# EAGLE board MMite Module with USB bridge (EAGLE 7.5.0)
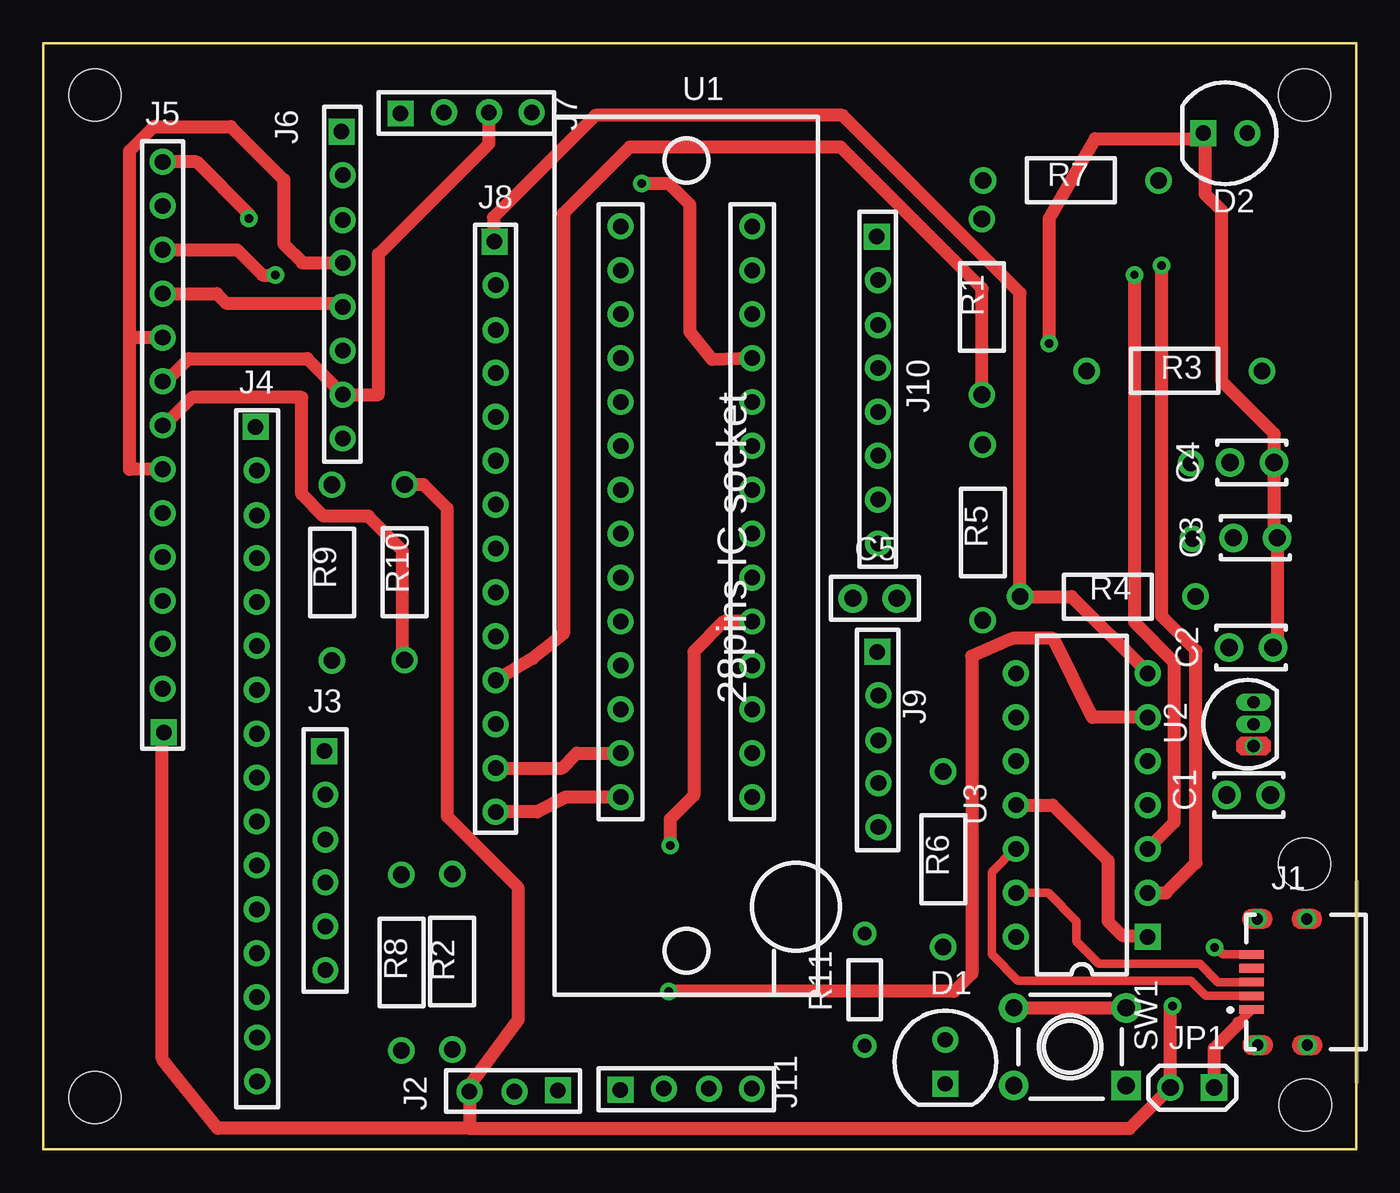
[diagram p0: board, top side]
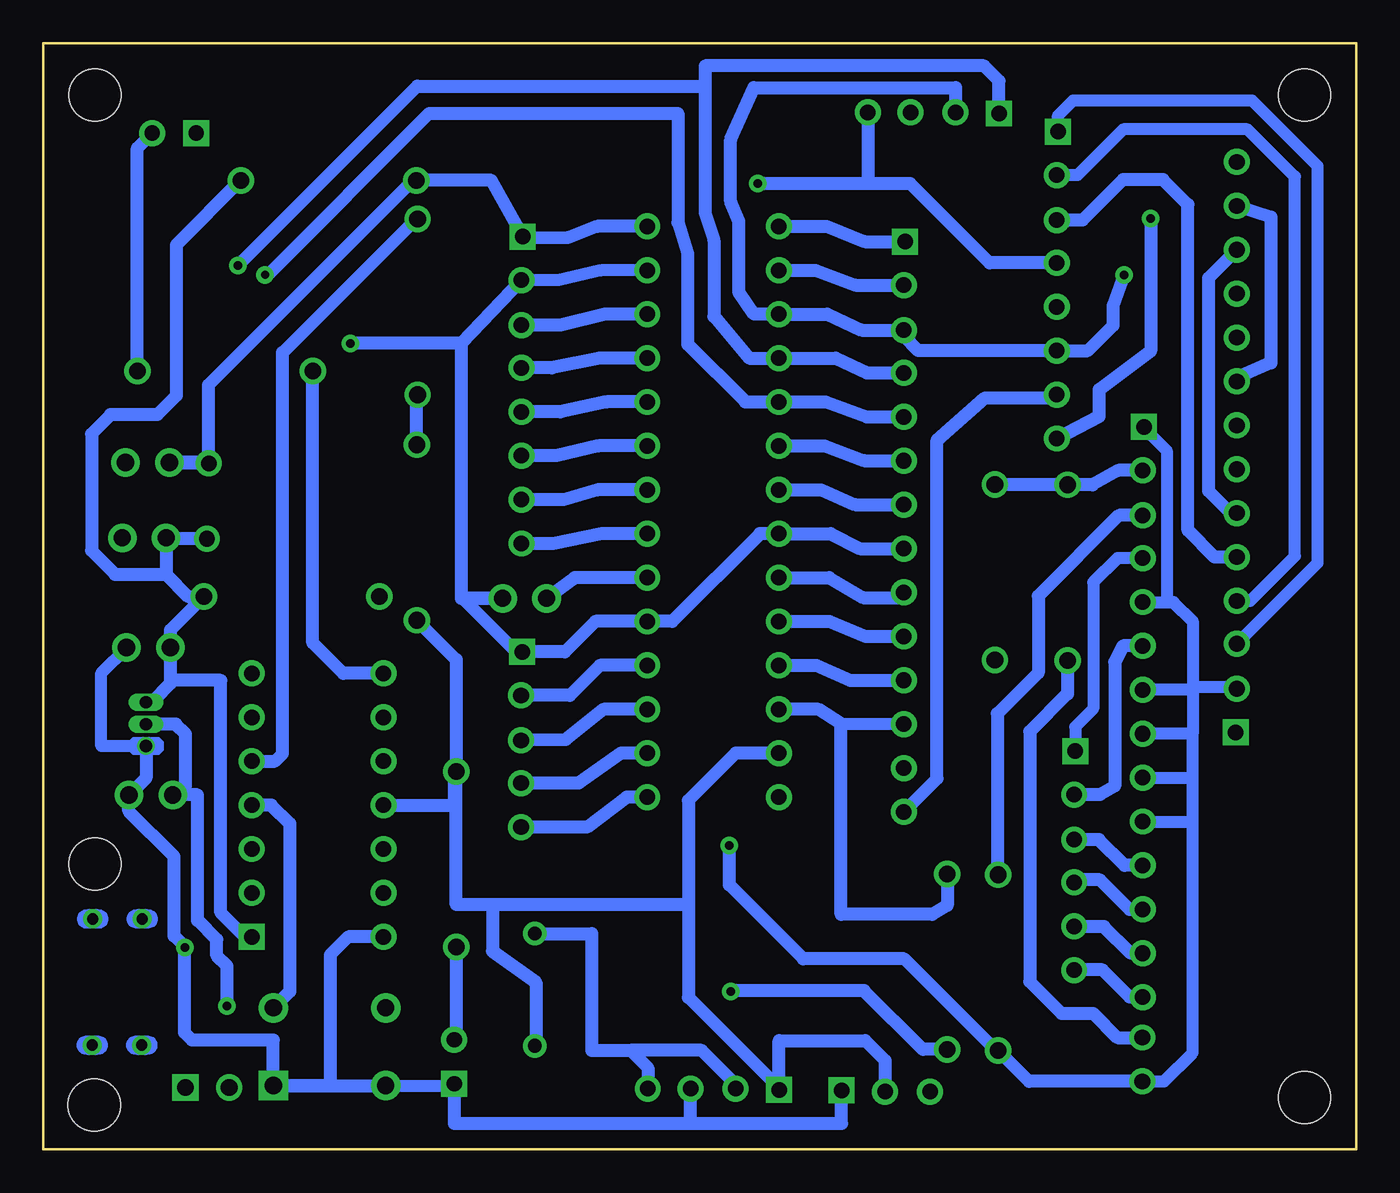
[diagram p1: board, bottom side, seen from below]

Size 76 x 64 mm. Coordinates in mm from the lower left corner, seen from the top.
Outline: 0,64 76,64 76,0 0,0 0,64
Copper layers (1*16): Top 0.035mm / dielectric 1.5mm / Bottom 0.035mm
Design rules "default *": minimum track width 10mil, minimum drill 0.61mm, track to track 8mil, track to pad 8mil, pad to pad 8mil, via to via 8mil, smd to smd 8mil, copper to edge 40mil, drill to drill 8mil, minimum pad ring 0mil, minimum via ring 8mil, stop-mask expansion 4mil, vias tented up to drill 19mil, thermal gap 10mil
Net classes: 0 Default: width 0.5 mm, clearance 0.33 mm
Holes 3 mm at 73.05,2.58 3,3 3,61 73,61 73,16.5

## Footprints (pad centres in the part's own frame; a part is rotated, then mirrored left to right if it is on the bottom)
CAP-2.54/4x2.5 = drill 1 pad 1.65: 1 -1.27,0; 2 1.27,0
CAP-2.54/5.1x2.5 = drill 1 pad 1.65: 1 -1.27,0; 2 1.27,0
LED-5Cil_Red = drill 0.889 pad 1.5 square: 1 -1.27,0 | drill 0.889 pad 1.5: 2 1.27,0
LED-5Cil_Green = drill 0.889 pad 1.5 square: 1 -1.27,0 | drill 0.889 pad 1.5: 2 1.27,0
Mini_USB_51387-578 = smd 0.5 x 1.4: 1 -1.6,1.75; 2 -0.8,1.75; 3 0,1.75; 4 0.8,1.75; 5 1.6,1.75 | drill 0.65 pad 1.1: 6 -3.65,1.396; 7 3.648,1.421; 8 -3.65,-1.472; 9 3.647,-1.447
CON3F = drill 0.9 pad 1.5 square: 1 -0.033,2.561 | drill 0.9 pad 1.5: 2 0.033,0.043; 3 0.033,-2.561
CON6F = drill 0.9 pad 1.5 square: 1 -0.033,6.339 | drill 0.9 pad 1.5: 2 0.033,3.821; 3 0.033,1.217; 4 0.033,-1.259; 5 0.033,-3.799; 6 0.033,-6.339
CON16F = drill 0.9 pad 1.5 square: 1 -0.044,18.937 | drill 0.9 pad 1.5: 2 0.022,16.419; 3 0.022,13.815; 4 0.022,11.339; 5 0.022,8.799; 6 0.022,6.259; 7 0.022,3.719; 8 0.022,1.179; 9 0.022,-1.361; 10 0.022,-3.901; 11 0.022,-6.441; 12 0.022,-8.981; 13 0.022,-11.521; 14 0.022,-14.061; 15 0.044,-16.397; 16 0.044,-18.937
CON14F = drill 0.9 pad 1.5 square: 1 -0.033,16.499 | drill 0.9 pad 1.5: 2 0.033,13.981; 3 0.033,11.377; 4 0.033,8.901; 5 0.033,6.361; 6 0.033,3.821; 7 0.033,1.281; 8 0.033,-1.259; 9 0.033,-3.799; 10 0.033,-6.339; 11 0.033,-8.879; 12 0.033,-11.419; 13 0.033,-13.959; 14 0.033,-16.499
CON8F = drill 0.9 pad 1.5 square: 1 -0.033,8.879 | drill 0.9 pad 1.5: 2 0.033,6.361; 3 0.033,3.757; 4 0.033,1.281; 5 0.033,-1.259; 6 0.033,-3.799; 7 0.033,-6.339; 8 0.033,-8.879
CON4F = drill 0.9 pad 1.5 square: 1 -0.033,3.799 | drill 0.9 pad 1.5: 2 0.033,1.281; 3 0.033,-1.323; 4 0.033,-3.799
CON5F = drill 0.9 pad 1.5 square: 1 -0.033,5.069 | drill 0.9 pad 1.5: 2 0.033,2.551; 3 0.033,-0.053; 4 0.033,-2.529; 5 0.033,-5.069
JMP = drill 0.965 pad 1.524 square: C1 -1.27,0 | drill 0.965 pad 1.524: C2 1.27,0
Pad = drill 0.9 pad 1.5: 1 0,0
RES-10.16/5.1x2.5 = drill 0.965 pad 1.524: 1 -5.08,0; 2 5.08,0
RES-10.16/5.1x2.5_R3 = drill 0.965 pad 1.524: 1 -5.08,0; 2 5.08,0
RES-6.5/3.4x1.9 = drill 0.8 pad 1.35: 1 -3.25,0; 2 3.25,0
B3F-1 = drill 1 pad 1.7 square: 1 -3.25,2.25 | drill 1 pad 1.7: 2 3.25,2.25; 3 -3.25,-2.25; 4 3.25,-2.25
28pins_ZIF_pattern = drill 0.9 pad 1.5: 1 -3.81,17.78; 2 -3.81,15.24; 3 -3.81,12.7; 4 -3.81,10.16; 5 -3.81,7.62; 6 -3.81,5.08; 7 -3.81,2.54; 8 -3.81,0; 9 -3.81,-2.54; 10 -3.81,-5.08; 11 -3.81,-7.62; 12 -3.81,-10.16; 13 -3.81,-12.7; 14 -3.81,-15.24; 15 3.81,-15.24; 16 3.81,-12.7; 17 3.81,-10.16; 18 3.81,-7.62; 19 3.81,-5.08; 20 3.81,-2.54; 21 3.81,0; 22 3.81,2.54; 23 3.81,5.08; 24 3.81,7.62; 25 3.81,10.16; 26 3.81,12.7; 27 3.81,15.24; 28 3.81,17.78
TO-92 = drill 0.7 pad 1: 1 -1.27,0 | drill 0.7 pad 1 long: 2 0,0; 3 1.27,0
DIP-14 = drill 0.9 pad 1.5 square: 1 -3.81,7.62 | drill 0.9 pad 1.5: 2 -3.81,5.08; 3 -3.81,2.54; 4 -3.81,0; 5 -3.81,-2.54; 6 -3.81,-5.08; 7 -3.81,-7.62; 8 3.81,-7.62; 9 3.81,-5.08; 10 3.81,-2.54; 11 3.81,0; 12 3.81,2.54; 13 3.81,5.08; 14 3.81,7.62

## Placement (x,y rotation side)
C1  10uF  [CAP-2.54/4x2.5]  69.77,20.51 0 top
C2  10uF  [CAP-2.54/4x2.5]  69.91,29.04 0 top
C3  100nF  [CAP-2.54/4x2.5]  70.15,35.39 0 top
C4  100nF  [CAP-2.54/4x2.5]  69.96,39.74 0 top
C5  47uF-16V Tan  [CAP-2.54/5.1x2.5]  48.14,31.88 0 top
D1  RED  [LED-5Cil_Red]  52.21,5.07 90 top
D2  GREEN  [LED-5Cil_Green]  68.42,58.79 0 top
J1  MINI USB  [Mini_USB_51387-578]  71.69,9.68 90 top
J2  HEADER 3F  [CON3F]  27.23,3.38 270 top
J3  HEADER 6F  [CON6F]  16.3,16.71 0 top
J4  HEADER 16F  [CON16F]  12.34,22.87 0 top
J5  HEADER 14F  [CON14F]  6.95,40.63 180 top
J6  HEADER 8F  [CON8F]  17.3,50.01 0 top
J7  HEADER 4F  [CON4F]  24.48,59.96 90 top
J8  HEADER 14F  [CON14F]  26.15,36.02 0 top
J9  HEADER 5F  [CON5F]  48.31,23.71 0 top
J10  HEADER 8F  [CON8F]  48.28,43.93 0 top
J11  HEADER 4F  [CON4F]  37.21,3.48 90 top
JP1  JUMPER  [JMP]  66.51,3.58 180 top
Pad1  PAD  [Pad]  66.41,39.69 0 top
Pad2  PAD  [Pad]  66.53,35.33 0 top
R1  1K5  [RES-10.16/5.1x2.5]  54.33,48.74 270 top
R2  1K5  [RES-10.16/5.1x2.5]  23.67,10.86 90 top
R3  1K  [RES-10.16/5.1x2.5_R3]  65.47,45.04 0 top
R4  10K  [RES-10.16/5.1x2.5_R3]  61.62,31.98 180 top
R5  10K  [RES-10.16/5.1x2.5]  54.38,35.69 90 top
R6  1K5  [RES-10.16/5.1x2.5]  52.1,16.78 270 top
R7  10R  [RES-10.16/5.1x2.5_R3]  59.48,56.06 180 top
R8  1K8  [RES-10.16/5.1x2.5]  20.74,10.81 270 top
R9  1K8  [RES-10.16/5.1x2.5]  16.71,33.37 270 top
R10  18R  [RES-10.16/5.1x2.5]  20.92,33.39 270 top
R11  100K  [RES-6.5/3.4x1.9]  47.55,9.24 90 top
SW1  SWITCH  [B3F-1]  59.43,5.94 180 top
U1  28pins ZIF  [28pins_ZIF_pattern]  37.23,35.62 0 top
U2  MCP1700-33  [TO-92]  70.05,24.61 90 top
U3  PIC16F1455  [DIP-14]  60.11,19.92 180 top

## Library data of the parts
C1-C4 = common; DESCRIPTION: Non-polarized
C5 = common; ATTR_1: Electrolytic; DESCRIPTION: Polarized
D1 D2 = common; DESCRIPTION: LED
J1 J2 J7 J9 J11 = common; DATASHEET: http://datasheets.diptrace.com/con_board_in/510221400_sd.pdf; MANUFACTURER: Molex
J3 J5 J8 J10 JP1 Pad1 Pad2 = common
J4 = common; DATASHEET: http://datasheets.diptrace.com/con_board_in/DF4.pdf; MANUFACTURER: Hirose
J6 = common; DATASHEET: http://datasheets.diptrace.com/con_board_in/510150300_sd.pdf; MANUFACTURER: Molex
R1-R11 = common; DESCRIPTION: Fixed Resistor
SW1 = common; ATTR_1: 2 Positions; DESCRIPTION: DIP Switch
U1 = common; MANUFACTURER: MICROMITE
U2 = common; DATASHEET: http://datasheets.diptrace.com/microchip/22008d.pdf; MANUFACTURER: Microchip
U3 = common; DATASHEET: http://datasheets.diptrace.com/microchip/21203Q.pdf; MANUFACTURER: Microchip

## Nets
Net_0: J8.1 R4.2 U1.1 U3.7
Net_1: C1.2 C2.2 C3.2 C4.2 C5.2 D1.1 D2.1 J1.5 J2.1 J4.1 J4.5 J4.7 J4.8 J4.9 J4.10 J4.16 J5.2 J8.8 J9.1 J10.2 J11.3 R8.2 SW1.1 SW1.2 U1.8 U1.19 U1.27 U2.1 U3.14
Net_2: C2.1 C3.1 J2.2 J8.13 J11.1 Pad2.1 R4.1 R5.1 R6.1 R7.1 R11.1 U1.13 U2.3 U3.1 U3.11
Net_3: J7.1 J8.4 U1.4 U3.2
Net_4: J8.5 U1.5 U3.3
Net_5: SW1.3 SW1.4 U3.4
Net_6: R1.1 U3.5
Net_7: J8.11 R1.2 R5.2 U1.11
Net_8: R2.1 U3.6
Net_9: J8.12 R2.2 U1.12
Net_10: R3.1 U3.8
Net_11: J1.3 U3.13
Net_12: D2.2 R3.2
Net_13: J1.2 U3.12
Net_14: C1.1 J2.3 J4.2 J5.1 JP1.C2 R9.1 R10.1 U2.2
Net_15: C5.1 U1.20
Net_16: D1.2 R6.2
Net_17: C4.1 J10.1 Pad1.1 R7.2 U1.28
Net_18: J3.1 J4.4
Net_19: J4.3 R8.1
Net_20: J11.2 J11.4 R11.2
Net_21: J3.6 J4.14
Net_22: J3.5 J4.13
Net_23: J3.4 J4.12
Net_24: J3.3 J4.11
Net_25: J3.2 J4.6
Net_26: J4.15 R9.2
Net_27: J9.2 U1.18
Net_28: J9.3 U1.17
Net_29: J9.4 U1.16
Net_30: J9.5 U1.15
Net_31: J10.3 U1.26
Net_32: J5.7 J5.10 J6.4 J7.4 J10.4 U1.25
Net_33: J10.5 U1.24
Net_34: J10.6 U1.23
Net_35: J10.7 U1.22
Net_36: J10.8 U1.21
Net_37: J8.2 U1.2
Net_38: J5.6 J5.12 J6.6 J7.2 J8.3 U1.3
Net_39: J8.6 U1.6
Net_40: J8.7 U1.7
Net_42: J8.9 U1.9
Net_43: J8.10 U1.10
Net_44: J5.9 J5.13 J6.7 J7.3 J8.14 U1.14
Net_45: J5.8 R10.2
Net_46: J1.1 JP1.C1
Net_49: J5.14 J6.8
Net_50: J5.11 J6.5
Net_51: J5.5 J6.3
Net_52: J5.4 J6.2
Net_53: J5.3 J6.1

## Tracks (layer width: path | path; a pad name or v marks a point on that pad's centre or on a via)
Net_0
  Top 0.75: J8.1 26.06,52.42 26.06,53.92 31.97,59.83 46.26,59.83 56.54,49.55 R4.2 59.52,31.98 63.92,27.58 U3.7
  Bottom 0.75: U1.1 30.64,53.4 28.45,52.52 J8.1
Net_1  (via drill 0.49 pad 1.02)
  Top 0.5: J1.5 68.28,11.28 67.89,11.67 v67.79,11.67
  Top 0.75: 52.21,3.69 D1.1 | v58.22,46.64 58.22,53.87 60.89,58.48 66.83,58.48 D2.1 67.24,58.8 67.24,55.27 68.19,54.33 68.19,44.47 71.23,41.43 C4.2 71.23,35.58 C3.2 71.42,29.28 C2.2 71.18,28.69 | U1.19 39.41,30.54 37.65,28.79 37.65,20.48 36.28,19.11 v36.28,17.57 | J4.7 12.36,26.65
  Bottom 0.7: J4.5 10.97,31.67 | 10.97,31.67 10.58,31.67 9.47,30.56 9.47,26.73 | 9.47,26.73 9.47,26.59 | 9.47,26.59 J4.7 | J5.2 6.92,26.73 9.47,26.73 | 9.47,26.59 9.47,24.05 | 9.47,24.05 J4.8 | J4.9 9.47,21.51 | 9.47,21.51 9.47,24.05 | J4.10 9.47,18.97 | 9.47,18.97 9.47,21.51 | J4.16 11.13,3.93 9.47,5.59 9.47,18.97 | U1.27 43.72,50.86 46.19,50.29 J10.2 | SW1.2 52.33,3.69 D1.1 | U2.1 72.64,23.34 72.64,27.57 C2.2 | J4.1 12.29,41.75 10.97,40.43 10.97,31.67
  Bottom 0.75: SW1.1 SW1.2 | SW1.2 | J10.2 51.8,46.64 | 51.8,46.64 v58.22,46.64 | 51.8,46.64 51.8,31.88 C5.2 51.73,31.88 48.63,28.78 J9.1 45.8,28.78 44.05,30.54 U1.19 39.6,30.54 34.52,35.62 U1.8 30.42,35.62 28.73,34.76 J8.8 | SW1.1 62.68,6.33 67.38,6.33 67.82,6.76 67.82,11.74 | 67.82,11.74 68.42,12.35 68.42,16.95 71.04,19.57 C1.2 70.05,21.5 U2.1 | D1.1 52.21,1.5 38.55,1.5 | 38.55,1.5 29.79,1.5 J2.1 | J11.3 38.55,3.51 38.55,1.5 | v67.79,11.67 67.82,11.74 | U3.14 58.35,12.3 59.39,11.26 59.39,3.69 SW1.1 | v36.28,17.57 36.28,15.3 32.01,11.02 26.16,11.02 20.86,5.73 R8.2 18.94,3.93 J4.16
Net_2
  Top 0.75: J8.13 30.02,22.06 30.88,22.92 U1.13 | U3.11 58.43,19.92 61.63,16.72 61.63,13.2 62.47,12.37 63.86,12.37 U3.1
  Bottom 0.75: 68.88,33.27 C3.1 68.83,35.33 Pad2.1 | 68.88,33.27 67.6,31.98 R4.1 68.64,30.04 C2.1 68.64,26.94 69.7,25.88 | R5.1 52.1,28.33 R6.1 | R7.1 68.3,52.32 68.3,43.6 69.39,42.51 72.1,42.51 73.2,41.4 73.2,34.64 71.83,33.27 68.88,33.27 | J2.2 27.27,5.15 28.41,6.3 33.41,6.3 J11.1 33.41,3.56 38.65,8.8 38.65,14.16 | U1.13 35.92,22.92 38.65,20.19 38.65,14.16 | 38.65,14.16 49.99,14.16 | 49.99,14.16 49.99,11.47 47.48,9.66 47.48,5.99 R11.1 | U3.1 64.33,12.3 65.72,13.69 65.72,27.13 68.45,27.13 69.7,25.88 | 69.7,25.88 U2.3 69.7,25.88 | 49.99,14.16 52.1,14.16 R6.1 | U3.11 52.19,19.92 52.19,21.86 R6.1
Net_3  (via drill 0.49 pad 1.02)
  Top 0.75: U3.2 64.98,14.84 66.72,16.58 66.72,28.88 64.74,30.85 v64.74,51.13
  Bottom 0.75: J8.4 28.33,44.92 30.12,45.78 U1.4 35.15,45.78 37.18,48.2 37.18,52.61 37.69,54.17 37.69,61.52 | J7.1 20.68,61.81 21.55,62.69 37.69,62.69 37.69,61.52 | v64.74,51.13 54.35,61.52 37.69,61.52
Net_4  (via drill 0.49 pad 1.02)
  Top 0.75: v63.16,50.6 63.16,30.52 65.45,28.23 65.45,18.9 U3.3
  Bottom 0.75: J8.5 28.34,42.38 30.7,43.24 U1.5 35.37,43.24 38.7,46.58 38.7,51.85 39.26,53.64 39.26,59.95 53.66,59.95 63.11,50.49 v63.16,50.6
Net_5
  Top 0.75: SW1.4 | SW1.4 SW1.3
  Bottom 0.75: SW1.3 61.72,9.15 61.72,18.84 62.8,19.92 U3.4
Net_6
  Bottom 0.75: U3.5 62.59,22.46 62.14,22.9 62.14,46.1 54.41,53.82 R1.1
Net_7
  Top 0.75: R1.2 54.33,49.82 46.17,57.98 33.95,57.98 30.11,54.15 30.11,29.84 28.33,28.4 J8.11
  Bottom 0.75: U1.11 31.24,28 29.28,27.14 J8.11 | R5.2 54.38,43.66 R1.2
Net_8  (via drill 0.49 pad 1.02)
  Top 0.75: U3.6 60.73,25 58.46,29.56 56.12,29.56 53.74,28.53 53.74,10.16 52.73,9.14 v36.2,9.14
  Bottom 0.75: R2.1 25.07,5.78 28.48,9.19 36.2,9.19 v36.2,9.14
Net_9
  Bottom 0.7: J8.12 29.66,24.6 29.82,24.45
  Bottom 0.75: R2.2 23.67,14.12 24.55,13.6 29.82,13.6 29.82,24.45 29.82,24.62 31.12,25.46 U1.12
Net_10
  Bottom 0.75: U3.8 58.63,27.54 60.39,29.3 R3.1
Net_11
  Top 0.5: U3.13 58.17,14.84 59.8,13.2 59.8,12.03 61.11,10.73 66.95,10.73 68,9.68 J1.3
Net_12
  Bottom 0.75: R3.2 70.55,57.93 D2.2
Net_13
  Top 0.5: U3.12 56.25,17.38 54.9,16.04 54.9,11.28 56.42,9.77 66.42,9.77 67.3,8.88 J1.2
Net_14  (via drill 0.49 pad 1.02)
  Top 0.75: J2.3 | J2.3 24.67,1.22 | 24.67,1.22 10.1,1.22 6.89,5.23 6.89,23.68 J5.1 | R10.1 21.99,38.48 23.38,37.09 23.38,19.26 27.48,15.16 27.48,7.47 24.56,3.54 J2.3 | J2.3 | v65.36,8.3 65.23,8.17 JP1.C2 62.88,1.22 24.67,1.22
  Bottom 0.75: 20.49,38.45 R10.1 | R10.1 | J4.2 13.79,39.29 15.27,38.45 R9.1 16.81,38.48 R10.1 | U2.2 68.33,24.61 67.76,24.04 67.76,21.02 68.5,20.28 C1.1 67.07,20.51 67.07,13.24 65.95,12.13 65.95,11.21 65.36,10.62 v65.36,8.3
Net_15
  Bottom 0.75: U1.20 45.24,33.08 47.11,31.7 C5.1
Net_16
  Bottom 0.75: R6.2 52.1,6.5 52.21,6.5 D1.2
Net_17
  Bottom 0.75: J10.1 48.16,52.73 | 48.16,52.73 50.05,56.06 R7.2 54.4,56.27 66.45,44.22 66.45,39.75 C4.1 68.64,39.69 Pad1.1 | U1.28 43.95,53.4 45.62,52.76 48.16,52.73
Net_18
  Bottom 0.7: J4.4 13.81,34.21 15.22,32.8 15.22,25.5 16.27,24.45 J3.1
Net_19
  Bottom 0.75: J4.3 13.74,36.69 18.41,32.01 18.41,27.57 20.78,25.21 20.78,15.93 R8.1
Net_20
  Bottom 0.75: R11.2 44.26,12.49 44.26,5.73 42.02,5.73 | 42.02,5.73 41.01,4.72 J11.4 | J11.2 35.93,3.76 37.89,5.73 42.02,5.73
Net_21
  Bottom 0.75: J4.14 13.12,8.81 14.7,10.38 16.32,10.38 J3.6
Net_22
  Bottom 0.75: J4.13 13.06,11.35 14.6,12.9 16.32,12.9 J3.5
Net_23
  Bottom 0.75: J4.12 13.12,13.89 14.83,15.6 16.18,15.6 J3.4
Net_24
  Bottom 0.75: J4.11 13.4,16.43 14.89,17.92 J3.3
Net_25
  Bottom 0.75: J4.6 13.5,29.13 13.98,28.19 13.98,21.02 14.84,20.53 J3.2
Net_26
  Bottom 0.75: R9.2 16.71,26.35 18.9,24.17 18.9,9.71 17.06,7.87 15.23,7.87 13.83,6.47 J4.15
Net_27
  Bottom 0.75: U1.18 43.77,28 45.51,26.27 J9.2
Net_28
  Bottom 0.75: U1.17 43.58,25.46 45.76,23.71 J9.3
Net_29
  Bottom 0.75: U1.16 42.54,22.92 45.01,21.19 J9.4
Net_30
  Bottom 0.75: U1.15 42.23,20.38 44.53,18.65 J9.5
Net_31
  Bottom 0.75: U1.26 43.49,48.32 46.04,47.69 J10.3
Net_32  (via drill 0.49 pad 1.02)
  Top 0.75: U1.25 38.73,45.69 37.43,47.31 37.43,54.66 36.21,55.88 v34.65,55.88 | J5.10 5,46.97 | 5,46.97 5,57.77 6.41,59.18 10.86,59.18 13.93,56.11 13.93,52.37 15.01,51.29 J6.4 | J5.7 5,39.35 5,46.97
  Bottom 0.75: U1.25 43.8,45.78 46.57,45.21 J10.4 | J6.4 21.22,51.29 25.82,55.88 28.28,55.88 | 28.28,55.88 v34.65,55.88 | J7.4 28.28,55.88
Net_33
  Bottom 0.75: U1.24 43.38,43.24 46.06,42.67 J10.5
Net_34
  Bottom 0.75: U1.23 43.87,40.7 46.28,40.13 J10.6
Net_35
  Bottom 0.75: U1.22 43.95,38.16 45.9,37.59 J10.7
Net_36
  Bottom 0.75: U1.21 43.67,35.62 46.48,35.05 J10.8
Net_37
  Bottom 0.75: U1.2 31.3,50.86 28.99,50 J8.2
Net_38  (via drill 0.49 pad 1.02)
  Top 0.75: J5.12 11.22,52.05 12.69,50.58 v13.44,50.58
  Bottom 0.75: J7.2 23.2,61.43 34.87,61.43 36.21,58.41 36.21,54.84 35.73,53.7 35.73,49.59 34.86,48.32 U1.3 30.61,48.32 28.63,47.4 J8.3 26.19,47.03 25.36,46.21 J6.6 15.54,46.21 14.08,47.67 14.08,48.81 13.4,50.66 v13.44,50.58 | J5.6 7.27,36.81 8.55,38.08 8.55,50.42 J5.12
Net_39
  Bottom 0.75: U1.6 30.77,40.7 28.5,39.84 J8.6
Net_40
  Bottom 0.75: U1.7 30.97,38.16 29.02,37.3 J8.7
Net_42
  Bottom 0.75: U1.9 30.52,33.08 28.55,31.92 26.49,31.92 J8.9
Net_43
  Bottom 0.75: U1.10 30.48,30.54 28.4,29.68 J8.10
Net_44
  Top 0.75: U1.14 30.24,20.38 28.59,19.52 J8.14 | J7.3 25.8,58.19 19.4,51.79 19.4,43.67 J6.7 17.33,43.7 15.28,45.75 8.43,45.75 7.12,44.43 J5.9
  Bottom 0.75: J8.14 24.26,21.45 24.26,41.04 21.48,43.48 17.33,43.48 J6.7 | J5.13 4.95,53.95 4.95,45.51 6.66,44.77 J5.9
Net_45
  Top 0.75: R10.2 | R10.2 20.8,28.54 20.8,34.64 18.81,36.63 16.22,36.63 14.96,37.89 14.96,43.51 8.63,43.51 7,41.89 J5.8
Net_46
  Top 0.5: 69.18,7.32 J1.1
  Top 0.75: JP1.C1 67.78,5.84 69.18,7.24 69.18,7.32
Net_49  (via drill 0.49 pad 1.02)
  Top 0.75: v11.9,53.87 11.9,54.1 8.87,57.13 J5.14
  Bottom 0.75: v11.9,53.87 11.9,46.2 14.89,43.95 14.89,42.4 J6.8
Net_50
  Top 0.75: J5.11 10.04,49.51 10.59,48.96 17.12,48.96 J6.5
Net_51
  Bottom 0.75: J5.5 8.2,34.27 9.74,35.81 9.74,54.66 11.19,56.11 13.51,56.11 15.85,53.76 J6.3
Net_52
  Bottom 0.7: J5.4 6.14,31.73 3.56,34.32 3.56,56.28 6.29,59.02 13.49,59.02 16.14,56.37 J6.2
  Bottom 0.75: J6.2 17.65,56.37
Net_53
  Bottom 0.7: J6.1 17.27,59.8 16.38,60.69 6.04,60.69 2.25,56.9 2.25,33.92 J5.3

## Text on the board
tDocu: SD | CS | CS | MO | MI | RESET | SCK | 1 | 1 | 28 | D/C | T-CLK(25) | T-CS | T-DIN(3) | T-DO(14) | 1 | T-IRQ | 21 | LCD ILI9341 MODULE | 1 | 19 | 14 | RS | EN | 15 | D4 | +5 | D5 | D6 | D7 | POWER I/O | EEPROM | /TEMP | LCD 16X2 MODULE | +5 | +3.3 | GND | +3.3 | I/O | GND | MM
